(* Logix 5000 DataType export Yaskawa_PLS_Switch; software revision 17.00 *)

TYPE Yaskawa_PLS_Switch :   // Structure of parameters needed for PLS switch operation using MPLS_Yaskawa v2.4.0
STRUCT
   FlagNumber : INT;   // Assigns a Flag number to the PLS output channel. Must be a physical output Flag 73-80, 88-90.
   OnPosition : REAL;   // If OnPosition < OffPosition output is ON between them. If OnPosition > OffPosition output is OFF between them and ON everywhere else.
   OffPosition : REAL;
   OnCompensation : INT;   // [msec]. Negative number turns output on SOONER, positive number turns output on LATER.
   OffCompensation : INT;   // [msec]
END_STRUCT
END_TYPE
